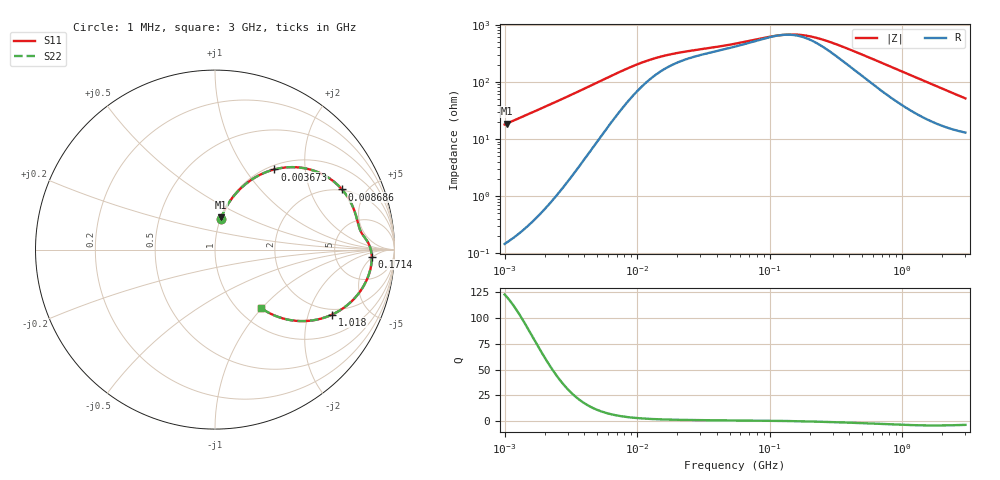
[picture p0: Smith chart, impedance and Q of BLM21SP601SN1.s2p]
! BLM21SP601SN1
# Hz S RI R 50
!Freq.(Hz) S11(Real) S11(Imag) S21(Real) S21(Imag) S12(Real) S12(Imag) S22(Real) S22(Imag)
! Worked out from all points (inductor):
!   401 points, 1 MHz to 3 GHz, reference 50 ohm
!   read as one part in series: L = 2.85 uH near 1.041 MHz
!   highest Q = 120 at 1.041 MHz (marker M1), where L = 2.84 uH
!   self-resonance near 123.5 MHz
!   S11 on the Smith chart (normalised r, x): 1 MHz: 1.00, +0.36; 3.673 MHz: 1.07, +1.38; 8.686 MHz: 1.95, +3.39; 171.4 MHz: 13, -4; 1.018 GHz: 1.76, -2.87; 3 GHz: 1.26, -0.99
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1000000  0.0322 0.1726  0.9678 -0.1726  0.9678 -0.1726  0.0322 0.1726
1040844  0.0348 0.1793  0.9652 -0.1793  0.9652 -0.1793  0.0348 0.1793
1522470  0.0722 0.2532  0.9278 -0.2532  0.9278 -0.2532  0.0722 0.2532
2097170  0.1308 0.3287  0.8692 -0.3287  0.8692 -0.3287  0.1308 0.3287
2775447  0.2135 0.396  0.7865 -0.396  0.7865 -0.396  0.2135 0.396
3673095  0.3305 0.4467  0.6695 -0.4467  0.6695 -0.4467  0.3305 0.4467
3823119  0.3497 0.4511  0.6503 -0.4511  0.6503 -0.4511  0.3497 0.4511
5481359  0.5319 0.4456  0.4681 -0.4456  0.4681 -0.4456  0.5319 0.4456
6969505  0.6378 0.397  0.3622 -0.397  0.3622 -0.397  0.6378 0.397
8686058  0.7074 0.3354  0.2926 -0.3354  0.2926 -0.3354  0.7074 0.3354
1.461624e7  0.7811 0.2032  0.2189 -0.2032  0.2189 -0.2032  0.7811 0.2032
2.459509e7  0.8022 0.1275  0.1978 -0.1275  0.1978 -0.1275  0.8022 0.1275
5.477226e7  0.8331 0.0688  0.1669 -0.0688  0.1669 -0.0688  0.8331 0.0688
1.148668e8  0.866 0.00766  0.134 -0.00766  0.134 -0.00766  0.866 0.00766
1.714156e8  0.8734 -0.0385  0.1266 0.0385  0.1266 0.0385  0.8734 -0.0385
2.094008e8  0.8728 -0.0653  0.1272 0.0653  0.1272 0.0653  0.8728 -0.0653
2.827291e8  0.8654 -0.1109  0.1346 0.1109  0.1346 0.1109  0.8654 -0.1109
4.480278e8  0.8321 -0.1956  0.1679 0.1956  0.1679 0.1956  0.8321 -0.1956
8.005644e8  0.7251 -0.3188  0.2749 0.3188  0.2749 0.3188  0.7251 -0.3188
1.017911e9  0.6516 -0.3625  0.3484 0.3625  0.3484 0.3625  0.6516 -0.3625
1.67892e9  0.4587 -0.3975  0.5413 0.3975  0.5413 0.3975  0.4587 -0.3975
3e9  0.2574 -0.3261  0.7426 0.3261  0.7426 0.3261  0.2574 -0.3261
